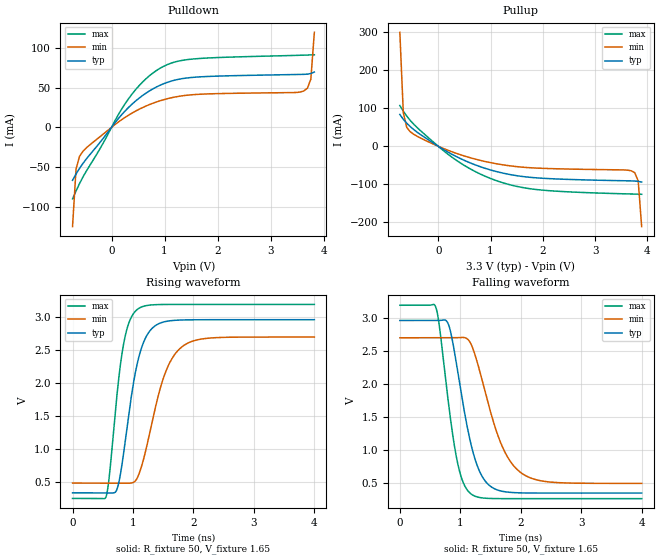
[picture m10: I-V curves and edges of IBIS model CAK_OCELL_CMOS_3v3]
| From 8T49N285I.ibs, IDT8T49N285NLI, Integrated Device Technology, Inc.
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[Model] CAK_OCELL_CMOS_3v3
Model_type   Output
Polarity   Non-Inverting
|   typ   min   max
C_comp   2pF   1.5pF   2.5pF
Vmeas = 1.65V
Rref = 50
Cref = 0
Vref = 1.65V
|   typ   min   max
[Voltage range]   3.3V   3.135V   3.465V
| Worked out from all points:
|   slope of the pulldown table from 0 to 0.495 V, typ, clamps not added: 14 ohm
|   slope of the pullup table from 0 to 0.495 V, typ, clamps not added: 13.5 ohm
|   rising waveform, R_fixture 50, V_fixture 1.65: 20-80 % time 276ps typ, 382ps min, 211ps max; typ from 0.339 V to 2.96 V
|   falling waveform, R_fixture 50, V_fixture 1.65: 20-80 % time 328ps typ, 454ps min, 255ps max; typ from 2.96 V to 0.339 V
[Pulldown]
|Voltage   I (typ)   I (min)   I (max)
|Note, modeling breaks down at 250mA and above.  This is well beyond the functional   |
|operating range of the device.  Should this scenario occur, catastrophic failure and   |
|possible damage to the device and/or board is of higher concern than the I-V curve   |
|behavior.  The IBIS checker will flag currents in excess of 10A with warnings.  Lines   |
|with currents in excess of 0.35 A have been commented out.  The points still remain|
|available to the user if the user desires to use them.   |
|-2.84000e+00   -2.18342e+01   -1.74861e+01   -2.67649e+01
|-2.38000e+00   -1.67175e+01   -1.36509e+01   -2.02266e+01
|-1.92000e+00   -1.16002e+01   -9.81576e+00   -1.36874e+01
|-1.46000e+00   -6.48170e+00   -5.98038e+00   -7.14724e+00
|-1.00000e+00   -1.36216e+00   -2.14477e+00   -6.05013e-01
|-9.99000e-01   -1.35103e+00   -2.13644e+00   -5.90785e-01
|-9.32920e-01   -6.15678e-01   -1.58547e+00   -1.41671e-01
|-8.66839e-01   -1.39919e-01   -1.03455e+00   -1.09705e-01
|-8.00759e-01   -7.88354e-02   -4.83652e-01   -9.97580e-02
-734.7mV  -66.59mA   -124.8mA   -89.95mA
-668.6mV  -58.64mA   -52.46mA   -80.04mA
-602.5mV  -51.57mA   -36.38mA   -70.7mA
-536.4mV  -45.18mA   -29.94mA   -62.18mA
322.6mV   25.15mA    15.4mA     36.14mA
586.9mV   40.13mA    24.92mA    57.09mA
917.3mV   53.03mA    33.49mA    74.43mA
1.512V    62.77mA    40.99mA    85.85mA
3.627V    66.71mA    45.82mA    90.85mA
3.693V    66.94mA    49.17mA    90.99mA
3.759V    67.73mA    60.6mA     91.14mA
3.825V    69.59mA    119.6mA    91.34mA
| 3.89095e+00   7.26618e-02   4.65706e-01   9.18943e-02
| 3.95703e+00   7.70381e-02   1.32521e+00   9.36022e-02
| 4.02311e+00   8.32626e-02   2.26645e+00   9.68439e-02
| 4.08920e+00   9.77618e-02   3.20770e+00   1.01650e-01
| 4.15528e+00   2.07471e-01   4.14908e+00   1.08027e-01
| 4.22136e+00   1.01792e+00   5.09063e+00   1.15660e-01
| 4.28744e+00   2.27449e+00   6.03236e+00   1.23032e-01
| 4.35352e+00   3.53161e+00   6.97425e+00   1.37138e-01
| 4.41960e+00   4.78899e+00   7.91633e+00   3.37460e-01
| 4.48568e+00   6.04663e+00   8.85859e+00   1.69666e+00
| 4.55176e+00   7.30454e+00   9.80103e+00   3.30464e+00
| 4.61784e+00   8.56273e+00   1.07437e+01   4.91299e+00
| 4.68392e+00   9.82120e+00   1.16865e+01   6.52170e+00
| 4.75000e+00   1.10799e+01   1.26295e+01   8.13079e+00
| 4.75100e+00   1.10990e+01   1.26438e+01   8.15514e+00
| 5.12080e+00   1.81486e+01   1.79250e+01   1.71669e+01
| 5.49060e+00   2.52080e+01   2.32134e+01   2.61912e+01
| 5.86040e+00   3.22784e+01   2.85101e+01   3.52280e+01
| 6.23020e+00   3.93607e+01   3.38170e+01   4.42714e+01
| 6.60000e+00   4.64524e+01   3.91358e+01   5.33146e+01
[Pullup]
|Voltage   I (typ)   I (min)   I (max)
|Note, modeling breaks down at 250mA and above.  This is well beyond the functional   |
|operating range of the device.  Should this scenario occur, catastrophic failure and   |
|possible damage to the device and/or board is of higher concern than the I-V curve   |
|behavior.  The IBIS checker will flag currents in excess of 10A with warnings.  Lines   |
|with currents in excess of 0.35 A have been commented out.  The points still remain|
|available to the user if the user desires to use them.   |
|-2.84000e+00   3.76971e+01   3.02376e+01   4.61593e+01
|-2.38000e+00   2.88981e+01   2.36451e+01   3.49141e+01
|-1.92000e+00   2.01037e+01   1.70553e+01   2.36741e+01
|-1.46000e+00   1.13159e+01   1.04719e+01   1.24414e+01
|-1.00000e+00   2.53397e+00   3.89369e+00   1.21369e+00
|-9.99000e-01   2.51488e+00   3.87939e+00   1.18929e+00
|-9.32920e-01   1.25355e+00   2.93464e+00   2.18725e-01
|-8.66839e-01   2.82239e-01   1.98975e+00   1.38859e-01
|-8.00759e-01   1.09379e-01   1.04415e+00   1.22843e-01
-734.7mV  83.53mA    299.1mA    106.9mA
-668.6mV  70.69mA    88.18mA    92.03mA
-602.5mV  60.53mA    49.54mA    79.23mA
-536.4mV  51.73mA    38.14mA    68.01mA
322.6mV   -25.41mA   -17.48mA   -34.57mA
719.1mV   -49.43mA   -34.12mA   -67.18mA
1.182V    -68.7mA    -47.53mA   -93.45mA
1.975V    -83.81mA   -57.81mA   -114.9mA
3.693V    -90.89mA   -64.39mA   -125.3mA
3.759V    -91.23mA   -69.4mA    -125.5mA
3.825V    -92.11mA   -91.04mA   -125.7mA
3.891V    -94mA      -210.8mA   -126mA
| 3.95703e+00   -9.70495e-02   -6.75177e-01   -1.26820e-01
| 4.02311e+00   -1.01334e-01   -1.22406e+00   -1.28839e-01
| 4.08920e+00   -1.08949e-01   -1.77316e+00   -1.32514e-01
| 4.15528e+00   -1.48643e-01   -2.32242e+00   -1.37667e-01
| 4.22136e+00   -5.15822e-01   -2.87181e+00   -1.43848e-01
| 4.28744e+00   -1.24821e+00   -3.42130e+00   -1.50145e-01
| 4.35352e+00   -1.98158e+00   -3.97088e+00   -1.58804e-01
| 4.41960e+00   -2.71518e+00   -4.52054e+00   -2.29366e-01
| 4.48568e+00   -3.44897e+00   -5.07027e+00   -9.38378e-01
| 4.55176e+00   -4.18293e+00   -5.62009e+00   -1.87630e+00
| 4.61784e+00   -4.91704e+00   -6.16997e+00   -2.81436e+00
| 4.68392e+00   -5.65127e+00   -6.71992e+00   -3.75252e+00
| 4.75000e+00   -6.38562e+00   -7.26994e+00   -4.69079e+00
| 4.75100e+00   -6.39674e+00   -7.27827e+00   -4.70499e+00
| 5.12080e+00   -1.05081e+01   -1.03576e+01   -9.95914e+00
| 5.49060e+00   -1.46224e+01   -1.34390e+01   -1.52184e+01
| 5.86040e+00   -1.87401e+01   -1.65231e+01   -2.04824e+01
| 6.23020e+00   -2.28625e+01   -1.96104e+01   -2.57530e+01
| 6.60000e+00   -2.69917e+01   -2.27023e+01   -3.10333e+01
[Ramp]
|   typ   min   max
dV/dt_r   1.576/0.275n   1.33/0.382n   1.767/0.211n
dV/dt_f   1.581/0.328n   1.332/0.454n   1.773/0.255n
R_load =   50.0000
[Rising Waveform]
R_fixture = 50
V_fixture = 1.65   |Vcc_typ
V_fixture_min = 1.5675 |Vcc_min
V_fixture_max = 1.7325 |Vcc_max
C_fixture = 0.0p
| Time   typ   min   max
0s        339.1mV    487mV      254.4mV
555.6ps   339.2mV    487mV      283.6mV
613.3ps   339.1mV    487mV      633.3mV
724.4ps   371.2mV    487mV      1.725V
831.1ps   850.7mV    487.2mV    2.526V
1.071ns   2.302V     566.3mV    3.12V
1.244ns   2.75V      1.113V     3.182V
1.507ns   2.93V      2.089V     3.196V
1.809ns   2.961V     2.553V     3.197V
4ns       2.965V     2.702V     3.197V
[Falling Waveform]
R_fixture = 50
V_fixture = 1.65   |Vcc_typ
V_fixture_min = 1.5675 |Vcc_min
V_fixture_max = 1.7325 |Vcc_max
C_fixture = 0.0p
| Time   typ   min   max
0s        2.965V     2.702V     3.197V
595.6ps   2.965V     2.702V     3.164V
657.8ps   2.965V     2.702V     2.852V
822.2ps   2.855V     2.702V     1.578V
986.7ps   2.02V      2.705V     675.2mV
1.173ns   1.095V     2.613V     329.7mV
1.453ns   479.4mV    1.731V     259.1mV
1.702ns   365.2mV    1.031V     254.8mV
1.978ns   343mV      667.7mV    254.5mV
4ns       339.1mV    487mV      254.4mV
